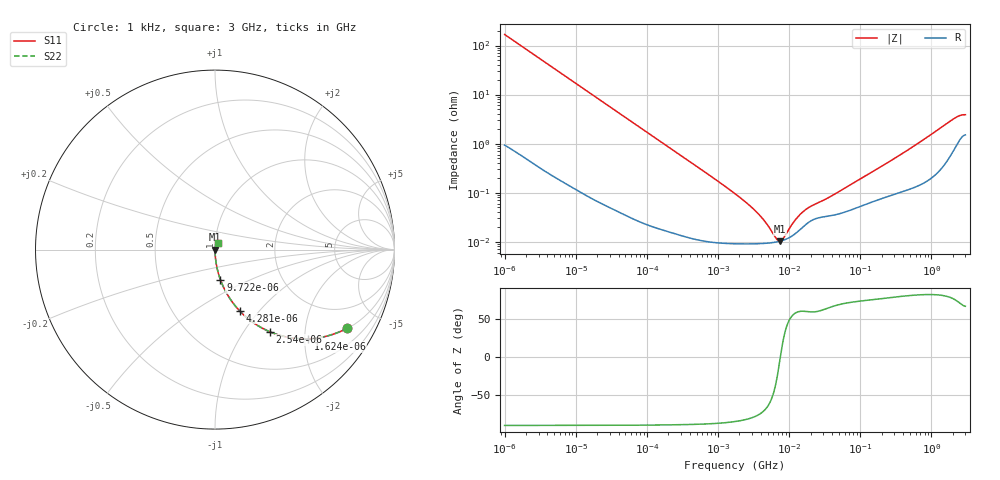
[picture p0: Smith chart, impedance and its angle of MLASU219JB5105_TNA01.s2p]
! MLASU219JB5105_TNA01  S-PARAMETER MODEL  ( Standard Model )
! Model Generated by TAIYO YUDEN Corporation (http://www.ty-top.com)
! Version 1.0
! TAIYO YUDEN Control No. 220601
! Copyright(c) 2010 TAIYO YUDEN CO.,LTD. All Rights Reserved.
! Product Description (link to TY-COMPAS)
! https://ds.yuden.co.jp/TYCOMPAS/or/detail?pn=MLASU219JB5105KTNA01&u=M
! Products Name : Multilayer Ceramic Capacitors
! Characteristics :
!  Capacitance : 1 [uF] , Rated Voltage : 50 [V] , TCC : X5R
!  Case Size : 2.0 x 1.25 / 0.079 x 0.049 [mm/inch] , Thickness : 0.85 / 0.033 [mm/inch]
!  (Conditions: Temperature = 25 [degC] , DC Bias Voltage = 0 [V])
! External Node Assignments :
!  1  o---| |---o  2
! GND o---------o GND
! Frequency Range : 1kHz  -  3GHz  [ 401 STEP ]
# MHZ S RI R 50
! Freq[MHz].  S11 Real  S11 Imag  S21 Real  S21 Imag  S12 Real  S12 Imag  S22 Real  S22 Imag
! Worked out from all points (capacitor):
!   401 points, 1 kHz to 3 GHz, reference 50 ohm
!   read as one part in series: C = 945 nF near 1.077 kHz
!   lowest |Z| = 10.3 mohm at 7.414 MHz (marker M1)
!   series resonance near 7.503 MHz, so ESL is about 480 pH
!   S11 on the Smith chart (normalised r, x): 1 kHz: 1.02, -3.36; 1.624 kHz: 1.01, -2.08; 2.54 kHz: 1.01, -1.33; 4.281 kHz: 1.00, -0.79; 9.722 kHz: 1.00, -0.35; 3 GHz: 1.03, +0.07
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0.001  0.7377 -0.4371  0.2623 0.4371  0.2623 0.4371  0.7377 -0.4371
0.001624  0.5185 -0.4968  0.4815 0.4968  0.4815 0.4968  0.5185 -0.4968
0.00254  0.3075 -0.4585  0.6925 0.4585  0.6925 0.4585  0.3075 -0.4585
0.004281  0.1365 -0.3403  0.8635 0.3403  0.8635 0.3403  0.1365 -0.3403
0.009722  0.0306 -0.169  0.9694 0.169  0.9694 0.169  0.0306 -0.169
0.01216  0.0201 -0.1367  0.9799 0.1367  0.9799 0.1367  0.0201 -0.1367
0.033275  0.00308 -0.0511  0.9969 0.0511  0.9969 0.0511  0.00308 -0.0511
0.147855  0.000318 -0.0116  0.9997 0.0116  0.9997 0.0116  0.000318 -0.0116
1.732051  9.16e-05 -0.00095  0.9999 0.00095  0.9999 0.00095  9.16e-05 -0.00095
3.651041  9.12e-05 -0.000365  0.9999 0.000365  0.9999 0.000365  9.12e-05 -0.000365
4.739869  9.3e-05 -0.000222  0.9999 0.000222  0.9999 0.000222  9.3e-05 -0.000222
6.629817  9.89e-05 -5.83e-05  0.9999 5.83e-05  0.9999 5.83e-05  9.89e-05 -5.83e-05
7.414467  0.000102 -5.56e-06  0.9999 5.56e-06  0.9999 5.56e-06  0.000102 -5.56e-06
8.291982  0.000108 4.74e-05  0.9999 -4.74e-05  0.9999 -4.74e-05  0.000108 4.74e-05
11.1738  0.000133 0.000193  0.9999 -0.000193  0.9999 -0.000193  0.000133 0.000193
13.46371  0.000165 0.000286  0.9998 -0.000286  0.9998 -0.000286  0.000165 0.000286
16.83921  0.00022 0.000388  0.9998 -0.000388  0.9998 -0.000388  0.00022 0.000388
21.06097  0.000275 0.000472  0.9997 -0.000472  0.9997 -0.000472  0.000275 0.000472
41.2049  0.000347 0.00082  0.9997 -0.00082  0.9997 -0.00082  0.000347 0.00082
256.0921  0.000873 0.00421  0.9991 -0.00421  0.9991 -0.00421  0.000873 0.00421
2066.299  0.00832 0.0309  0.9917 -0.0309  0.9917 -0.0309  0.00832 0.0309
3000  0.016 0.0348  0.984 -0.0348  0.984 -0.0348  0.016 0.0348
